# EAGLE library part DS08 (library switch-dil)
DIL/CODE SWITCH
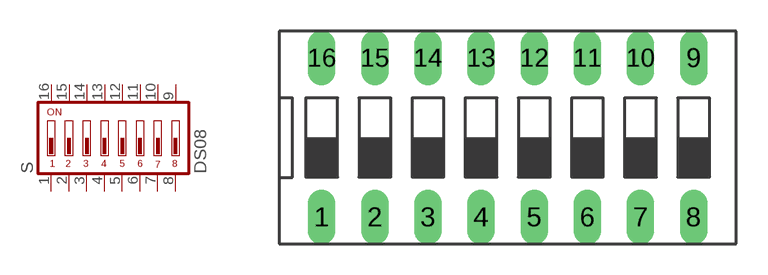
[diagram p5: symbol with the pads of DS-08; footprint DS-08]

Designator prefix S

## DS08 (MPN: DS08; OC_FARNELL: unknown; OC_NEWARK: 73J0071)  [DS-08]
1  1  pas
2  2  pas
3  3  pas
4  4  pas
5  5  pas
6  6  pas
7  7  pas
8  8  pas
9  9  pas
10  10  pas
11  11  pas
12  12  pas
13  13  pas
14  14  pas
15  15  pas
16  16  pas

## Footprint DS-08 (pad centres in mm)
DIL/CODE SWITCH Mors distributor Buerklin, 17G562
drill 0.813 long: 1 -8.89,-3.81; 2 -6.35,-3.81; 3 -3.81,-3.81; 4 -1.27,-3.81; 5 1.27,-3.81; 6 3.81,-3.81; 7 6.35,-3.81; 8 8.89,-3.81; 9 8.89,3.81; 10 6.35,3.81; 11 3.81,3.81; 12 1.27,3.81; 13 -1.27,3.81; 14 -3.81,3.81; 15 -6.35,3.81; 16 -8.89,3.81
